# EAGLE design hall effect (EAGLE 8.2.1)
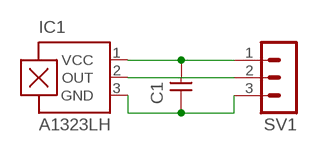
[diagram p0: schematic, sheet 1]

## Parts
C1  CAP-UNPOLARIZEDFAB  [C1206FAB]
IC1  A1323LH  [SOT23-W]
SV1  MA03-1  [MA03-1]

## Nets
N$1: C1.2 IC1.1(VCC) SV1.1
N$2: C1.1 IC1.3(GND) SV1.3
N$3: IC1.2(OUT) SV1.2

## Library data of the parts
C1 = fab:CAP-UNPOLARIZED
IC1 = allegro:A13*?: Linear Hall Effect Sensor ICs Continuous-Time Ratiometric High-Temperature Operation Programmable Linear with Analog Output A1302 -Replacement- UGN3503 Source: http://www.allegromicro.com/en/Products/Part_Numbers/1301/1301.pdf http://www.allegromicro.com/en/Products/Part_Numbers/1321/1321.pdf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; MF: ALLEGRO MICROSYSTEMS, INC.; MPN: A1323LLHLT-T; OC_FARNELL: 1651968; OC_NEWARK: 65K5152
SV1 = con-lstb:MA03-1: PIN HEADER; OC_FARNELL: unknown; OC_NEWARK: unknown

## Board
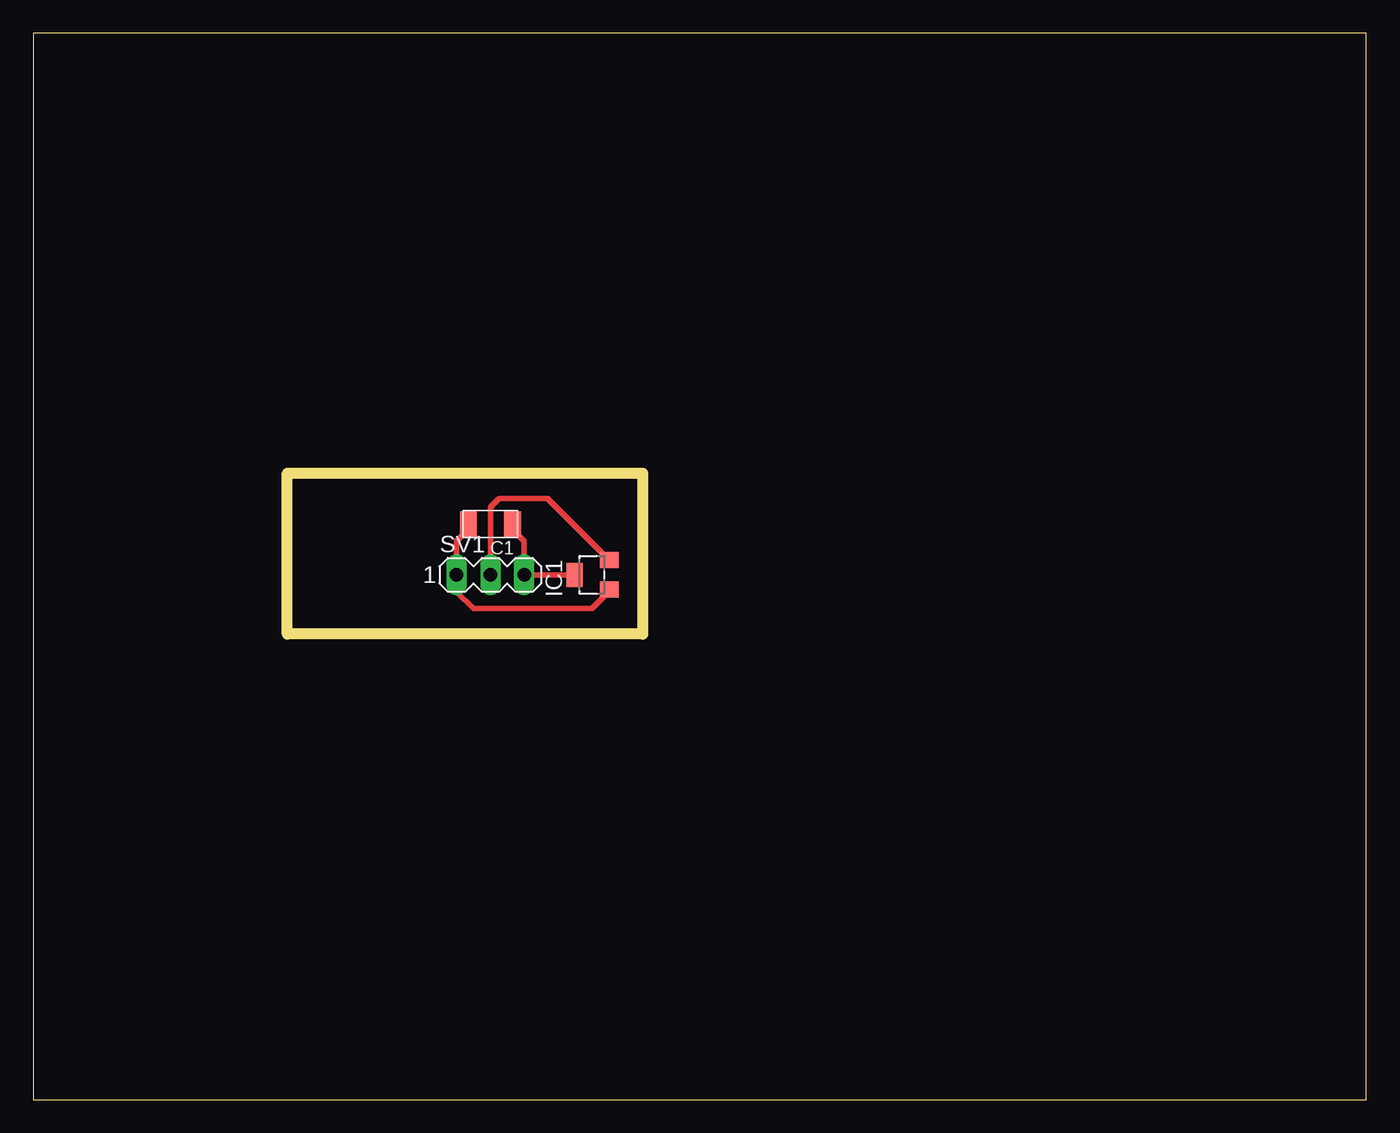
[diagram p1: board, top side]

Size 100 x 80 mm. Coordinates in mm from the lower left corner, seen from the top.
Outline: 0,0 100,0 100,80 0,80 0,0
Outline: 19.05,46.99 45.72,46.99 45.72,34.92 19.05,34.92 19.05,46.99
Copper layers (1*16): Top 0.035mm / dielectric 1.5mm / Bottom 0.035mm
Design rules "default": minimum track width 6mil, minimum drill 0.35mm, track to track 6mil, track to pad 6mil, pad to pad 6mil, via to via 6mil, smd to smd 6mil, copper to edge 40mil, drill to drill 6mil, minimum pad ring 10mil, minimum via ring 8mil, stop-mask expansion 4mil, vias tented up to drill 0mil, thermal gap 10mil

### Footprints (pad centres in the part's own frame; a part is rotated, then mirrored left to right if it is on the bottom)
C1206FAB = smd 1.27 x 1.905: 1 -1.651,0; 2 1.651,0
SOT23-W = smd 1.2 x 1.4: 1 -1.1,-1.3; 2 1.1,-1.3 | smd 1.8 x 1.2: 3 0,1.3
MA03-1 = drill 1.016 long: 1 -2.54,0; 2 0,0; 3 2.54,0

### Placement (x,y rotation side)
C1  34.29,43.18 180 top
IC1  41.91,39.37 90 top
SV1  34.29,39.37 0 top

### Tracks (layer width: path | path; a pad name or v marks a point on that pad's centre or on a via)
N$1
  Top 0.406: IC1.1 43.21,38.13 41.91,36.83 33.02,36.83 31.75,38.1 SV1.1 31.75,41.91 32.38,42.55 32.38,42.93 C1.2
N$2
  Top 0.406: C1.1 36.2,42.93 36.2,42.55 36.83,41.91 SV1.3 IC1.3
N$3
  Top 0.406: SV1.2 34.29,44.45 34.92,45.09 38.59,45.09 IC1.2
